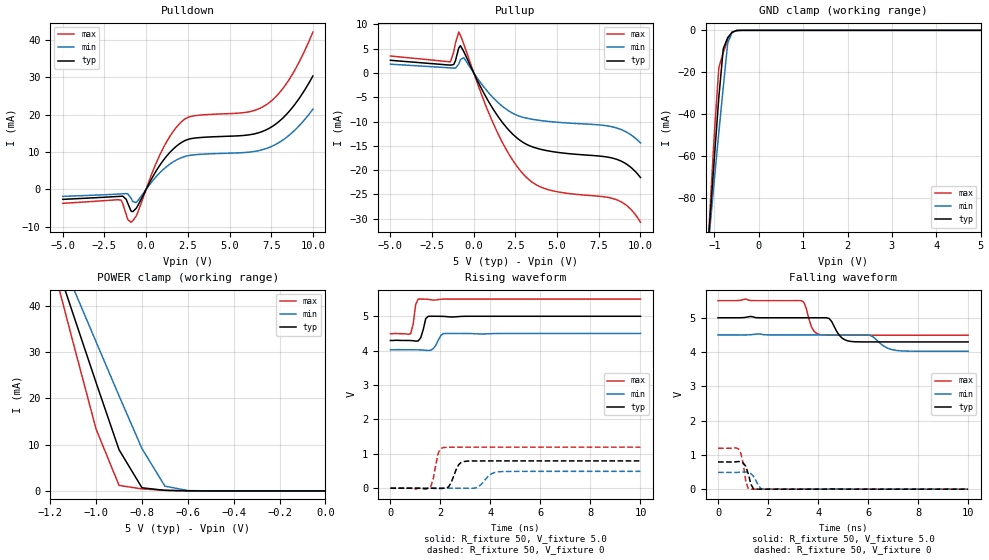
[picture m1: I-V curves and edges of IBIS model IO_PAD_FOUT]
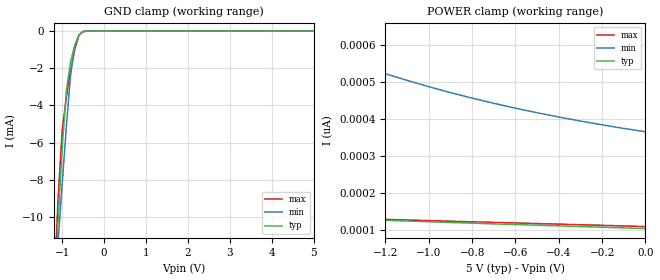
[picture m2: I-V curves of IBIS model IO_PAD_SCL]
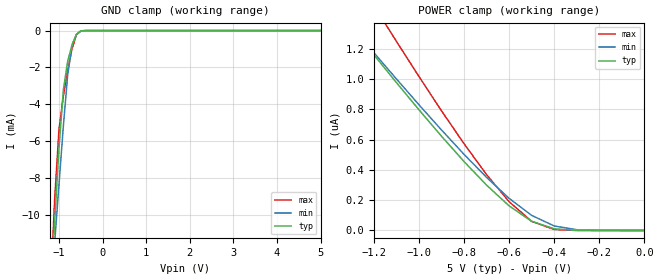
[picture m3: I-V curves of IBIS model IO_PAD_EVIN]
[IBIS Ver]   3.2
[Comment Char]   |_char
[File name]   rx8111ce_5v.ibs
[File Rev]   1.0
[Date]   2019/09/17 2:32:47
[Source]
[Notes]
[Disclaimer]
This information is for modeling purposes only, and is not guaranteed.
Property of SEIKO EPSON Corp.,
unauthorized reproduction and/or distribution is strictly prohibited.
[Copyright]
Copyright 2019, SEIKO EPSON Corp.
[Component]   T5462W0B
Si_location Pin
Timing_location Pin
[Manufacturer]   SEIKO EPSON Corp.
| RX-8111CE
[Package]
R_pkg   0.0m   0.0m   0.0m
L_pkg   0.0n   0.0n   0.0n
C_pkg   0.0p   0.0p   0.0p
[Pin] signal_name   model_name
1   VDD   POWER
2   VOUT   POWER
3   VBAT   POWER
4   FOUT   IO_PAD_FOUT
5   SCL   IO_PAD_SCL
6   EVIN   IO_PAD_EVIN
7   SDA   IO_PAD_SDA
8   VIO   POWER
9   GND   GND
10   /INT   IO_PAD_XINT
| Models and submodels in the file (5): IO_PAD_FOUT (3-state), IO_PAD_SCL (Input), IO_PAD_EVIN (Input), IO_PAD_SDA (I/O_open_drain), IO_PAD_XINT (Open_drain)
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[Model]   IO_PAD_FOUT
Model_type 3-state
Enable Active-High
Polarity Non-Inverting
Vmeas=2.50
C_comp   2.5p   2.0p   3.0p
[Temperature Range] 25   105   -40
[Voltage Range]   5.0   4.5   5.5
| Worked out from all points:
|   slope of the pulldown table from 0 to 0.75 V, typ, clamps not added: 126 ohm
|   slope of the pullup table from 0 to 0.75 V, typ, clamps not added: 149 ohm
|   GND clamp passes 1 mA (typ) near -0.60 V on its own axis
|   POWER clamp passes 1 mA (typ) near -0.80 V on its own axis
|   falling waveform, R_fixture 50, V_fixture 5.0: 20-80 % time 354ps typ, 503ps min, 257ps max; typ from 5 V to 4.29 V
|   falling waveform, R_fixture 50, V_fixture 0: 20-80 % time 185ps typ, 230ps min, 167ps max; typ from 0.793 V to 0 V
|   rising waveform, R_fixture 50, V_fixture 5.0: 20-80 % time 152ps typ, 215ps min, 119ps max; typ from 4.29 V to 5 V
|   rising waveform, R_fixture 50, V_fixture 0: 20-80 % time 269ps typ, 381ps min, 199ps max; typ from 0 V to 0.793 V
[Pullup]
-5V       2.598mA    1.801mA    3.488mA
-1.4V     1.602mA    1.04mA     2.29mA
-1.2V     1.734mA    995.3uA    4.356mA
-900mV    5.147mA    1.814mA    8.407mA
-600mV    4.408mA    3.126mA    5.954mA
1.2V      -7.642mA   -5.236mA   -10.62mA
2.1V      -11.76mA   -7.82mA    -16.67mA
3V        -14.38mA   -9.175mA   -20.93mA
4.5V      -16.07mA   -9.985mA   -24.05mA
8.6V      -17.81mA   -11.36mA   -26.14mA
9.4V      -19.36mA   -12.67mA   -28mA
10V       -21.52mA   -14.39mA   -30.72mA
[Pulldown]
-5V       -2.695mA   -1.899mA   -3.76mA
-1.5V     -1.871mA   -1.232mA   -2.909mA
-1.1V     -3.756mA   -1.223mA   -8.145mA
-900mV    -5.868mA   -2.416mA   -8.805mA
-600mV    -5.116mA   -3.564mA   -7.202mA
900mV     6.952mA    4.772mA    9.936mA
2V        12.16mA    8.239mA    17.55mA
2.7V      13.56mA    9.131mA    19.52mA
6.1V      14.53mA    9.907mA    20.68mA
7.3V      16.12mA    11.06mA    22.91mA
8.6V      20.95mA    14.55mA    29.52mA
10V       30.3mA     21.42mA    42.06mA
[GND Clamp]
-5V       -1.289A    -1.043A    -1.612A
-1.2V     -119.6mA   -117.1mA   -123.7mA
-1.1V     -89.89mA   -93.83mA   -85.8mA
-1V       -60.42mA   -70.86mA   -48.73mA
-900mV    -31.79mA   -48.51mA   -17.79mA
-800mV    -8.762mA   -26.99mA   -10.57mA
-700mV    -3.482mA   -6.087mA   -4.558mA
-600mV    -875.1uA   -938.3uA   -964.6uA
-500mV    -86.79uA   -136.7uA   -53.06uA
-400mV    -4.756uA   -14.79uA   -1.084uA
5V        63.88pA    6.455uA    39.96pA
[POWER Clamp]
-5V       627.4mA    509.9mA    781.1mA
-1.2V     53.06mA    55.67mA    50.97mA
-1.1V     38.19mA    43.92mA    32.03mA
-1V       23.39mA    32.21mA    13.34mA
-900mV    8.899mA    20.56mA    1.198mA
-800mV    681.2uA    9.149mA    429.9uA
-700mV    117.2uA    1.034mA    142uA
-600mV    22.79uA    76.25uA    23.1uA
0V        63.54pA    1.113nA    49.41pA
[Falling Waveform]
R_fixture=50
V_fixture=5.0
V_fixture_min=4.5
V_fixture_max=5.5
0s        5V         4.5V       5.5V
3.333ns   5V         4.5V       5.499V
3.838ns   5V         4.5V       4.608V
4.141ns   5V         4.5V       4.501V
4.444ns   4.977V     4.5V       4.493V
4.848ns   4.489V     4.5V       4.492V
5.253ns   4.316V     4.5V       4.492V
6.061ns   4.295V     4.492V     4.492V
7.172ns   4.295V     4.044V     4.492V
10ns      4.295V     4.024V     4.492V
[Falling Waveform]
R_fixture=50
V_fixture=0
V_fixture_min=0
V_fixture_max=0
0s        793.4mV    489.5mV    1.193V
808.1ps   805.6mV    490.2mV    1.178V
909.1ps   802.1mV    494.8mV    1.058V
1.01ns    763mV      499.2mV    734.5mV
1.111ns   664.1mV    500.2mV    224mV
1.212ns   439.3mV    488.6mV    10.14mV
1.414ns   12.91mV    379mV      74.07uV
1.616ns   264.6uV    106.9mV    -4.661uV
1.818ns   -9.787uV   3.8mV      -18.98uV
10ns      0V         0V         0V
[Rising Waveform]
R_fixture=50
V_fixture=5.0
V_fixture_min=4.5
V_fixture_max=5.5
0s        4.295V     4.024V     4.492V
808.1ps   4.294V     4.025V     4.493V
909.1ps   4.289V     4.024V     4.763V
1.01ns    4.277V     4.024V     5.343V
1.111ns   4.282V     4.024V     5.499V
1.212ns   4.375V     4.021V     5.5V
1.414ns   4.934V     4.01V      5.497V
1.515ns   4.999V     4.005V     5.492V
2.121ns   4.997V     4.499V     5.499V
10ns      5V         4.5V       5.5V
[Rising Waveform]
R_fixture=50
V_fixture=0
V_fixture_min=0
V_fixture_max=0
0s        0V         0V         0V
1.616ns   96.93uV    -1.137mV   51.94mV
1.919ns   -648.9uV   -11.19mV   1.033V
2.121ns   -2.477mV   -4.226mV   1.182V
2.323ns   37mV       -40.99uV   1.19V
2.727ns   680.2mV    7.872uV    1.192V
3.03ns    784.9mV    -1.033mV   1.193V
3.434ns   792.1mV    13.43mV    1.193V
4.343ns   793.3mV    476.9mV    1.193V
10ns      793.4mV    489.5mV    1.193V
[Ramp]
R_load=50
dV/dt_r   4.760E-1/2.599E-10   2.937E-1/3.667E-10   7.157E-1/1.807E-10
dV/dt_f   4.228E-1/3.439E-10   2.856E-1/5.027E-10   6.049E-1/2.422E-10
|[End   IO_PAD_FOUT
[Model]   IO_PAD_SCL
Model_type Input
Enable Active-High
Polarity Non-Inverting
Vinh=4.4
Vinl=0.9
C_comp   2.5p   2.0p   3.0p
[Temperature Range] 25   105   -40
[Voltage Range]   5.0   4.5   5.5
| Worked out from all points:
|   GND clamp passes 1 mA (typ) near -0.73 V on its own axis
[GND Clamp]
-5V       -174.9mA   -140.3mA   -216.1mA
-1.2V     -14.34mA   -14.53mA   -14.15mA
-1.1V     -10.3mA    -11.38mA   -9.069mA
-1V       -6.301mA   -8.235mA   -5.326mA
-900mV    -3.193mA   -5.118mA   -3.551mA
-800mV    -1.656mA   -2.372mA   -2.158mA
-700mV    -763.9uA   -783.6uA   -983.1uA
-600mV    -207.7uA   -205.2uA   -228.8uA
-500mV    -21.87uA   -34.9uA    -13.49uA
-300mV    -47.01nA   -341.4nA   -3.545nA
5V        104.2pA    416.4pA    99.8pA
[POWER Clamp]
-5V       237.5pA    2.814nA    8.229uA
-4.7V     224.1pA    2.464nA    4.117nA
-4.6V     220.3pA    2.356nA    227.2pA
-4.5V     216.1pA    2.252nA    183.3pA
-3V       167.6pA    1.122nA    157.6pA
-1.7V     136.7pA    631.2pA    136.9pA
-1.5V     132.7pA    583.1pA    133.6pA
-1.3V     128.6pA    540.9pA    130.5pA
-1.1V     124.4pA    503.5pA    127.2pA
-900mV    120.6pA    470.6pA    124pA
-500mV    113.1pA    416.4pA    117.6pA
0V        104.2pA    365.1pA    109.5pA
[Model]   IO_PAD_EVIN
Model_type Input
Enable Active-High
Polarity Non-Inverting
Vinh=4.4
Vinl=0.9
C_comp   2.5p   2.0p   3.0p
[Temperature Range] 25   105   -40
[Voltage Range]   5.0   4.5   5.5
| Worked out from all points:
|   GND clamp passes 1 mA (typ) near -0.73 V on its own axis
[GND Clamp]
-5V       -177.7mA   -142.7mA   -219.5mA
-1.2V     -14.52mA   -14.72mA   -14.31mA
-1.1V     -10.41mA   -11.52mA   -9.158mA
-1V       -6.363mA   -8.33mA    -5.355mA
-900mV    -3.212mA   -5.172mA   -3.552mA
-800mV    -1.657mA   -2.392mA   -2.158mA
-700mV    -764.4uA   -786.1uA   -983.6uA
-600mV    -208.1uA   -205.5uA   -229.1uA
-500mV    -22.03uA   -35.1uA    -13.63uA
-300mV    -50.63nA   -359nA     -4.13nA
5V        115.8pA    99.35nA    104.6pA
[POWER Clamp]
-5V       9.254uA    8.653uA    19.97uA
-1.3V     1.344uA    1.347uA    1.722uA
-1.2V     1.158uA    1.172uA    1.482uA
-1.1V     974.4nA    998.5nA    1.246uA
-900mV    620.9nA    662.1nA    788.4nA
-800mV    454nA      501.5nA    571.3nA
-700mV    298.5nA    349.4nA    368nA
-600mV    162nA      211.5nA    189.4nA
-500mV    60.49nA    99.34nA    59.91nA
-400mV    10.97nA    29.68nA    6.406nA
-300mV    904.7pA    5.083nA    296.2pA
0V        115pA      388.1pA    121.3pA
